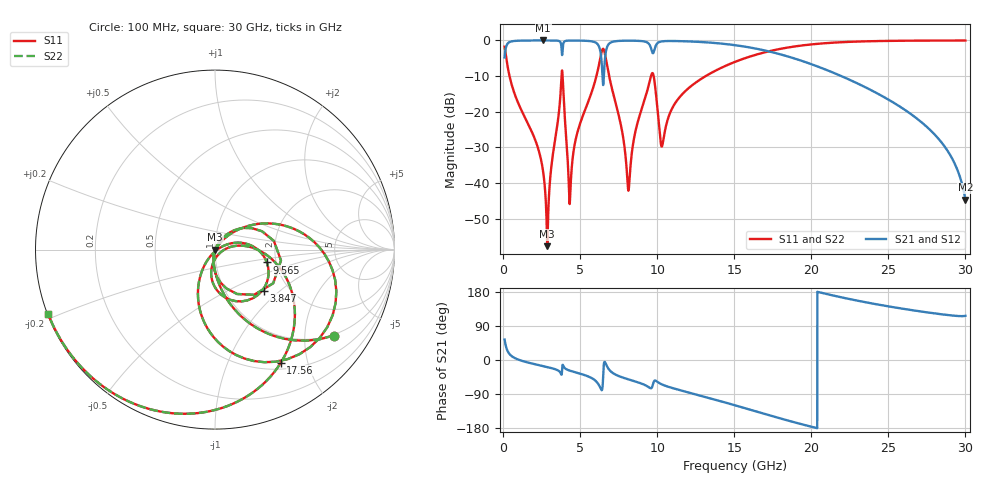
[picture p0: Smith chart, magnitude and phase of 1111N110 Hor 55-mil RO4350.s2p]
# GHz S MA R 50
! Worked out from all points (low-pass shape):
!   3201 points, 100 MHz to 30 GHz, reference 50 ohm
!   highest |S21| = -0.01 dB at 2.604 GHz (marker M1); lowest = -44.6 dB at 30 GHz (marker M2)
!   |S21| within 3 dB of the highest: 141.6 MHz to 3.807 GHz (3.665 GHz wide, 186 % of centre); 9.792 GHz to 17.18 GHz (7.388 GHz wide, 54.8 % of centre)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
!   lowest |S11| = -57.7 dB at 2.866 GHz (marker M3), VSWR 1.00, Z = 50.1 - j0.0687 ohm
!   |S11| at or under -10 dB: 419.5 MHz to 3.795 GHz (3.375 GHz wide, 160 % of centre); 6.882 GHz to 9.598 GHz (2.715 GHz wide, 33 % of centre); 9.772 GHz to 13.15 GHz (3.376 GHz wide, 29.5 % of centre)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
!   |S22| runs from -57.7 to 0.0 dB; largest |S21 - S12| = 0
!   S11 on the Smith chart (normalised r, x): 100 MHz: 0.97, -2.79; 3.847 GHz: 1.50, -0.79; 9.565 GHz: 1.78, -0.28; 17.56 GHz: 0.59, -1.58; 30 GHz: 0.00, -0.19
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0.1  0.8167 -35.9  0.5767 54.1  0.5767 54.1  0.8167 -35.9
0.585875  0.2293 -80.5  0.9728 9.4  0.9728 9.4  0.2293 -80.5
2.604125  0.01427 -101.9  0.9985 -16.2  0.9985 -16.2  0.01427 -101.9
2.86575  0.001308 -31.6  0.9984 -18.7  0.9984 -18.7  0.001308 -31.6
3.846844  0.3579 -40.1  0.6608 -16.8  0.6608 -16.8  0.3579 -40.1
4.332719  0.00527 -8.7  0.9945 -28.1  0.9945 -28.1  0.00527 -8.7
5.089563  0.07796 49.8  0.9923 -37.2  0.9923 -37.2  0.07796 49.8
6.15475  0.3876 21.1  0.875 -61.9  0.875 -61.9  0.3876 21.1
6.5285  0.7488 -51.2  0.2893 -16.0  0.2893 -16.0  0.7488 -51.2
6.874219  0.3226 -106.1  0.897 -25.0  0.897 -25.0  0.3226 -106.1
8.144969  0.007926 -42.1  0.9913 -51.3  0.9913 -51.3  0.007926 -42.1
9.565219  0.2977 -13.9  0.8185 -74.5  0.8185 -74.5  0.2977 -13.9
9.789469  0.3015 -70.6  0.7038 -56.5  0.7038 -56.5  0.3015 -70.6
10.06978  0.08501 -99.5  0.9326 -59.2  0.9326 -59.2  0.08501 -99.5
10.33141  0.03362 -31.6  0.9706 -64.9  0.9706 -64.9  0.03362 -31.6
11.59281  0.1732 6.5  0.9756 -80.9  0.9756 -80.9  0.1732 6.5
15.05  0.5004 -30.3  0.8576 -119.5  0.8576 -119.5  0.5004 -30.3
17.56347  0.7289 -59.8  0.6749 -149.2  0.6749 -149.2  0.7289 -59.8
20.03956  0.8807 -86.9  0.4615 -176.4  0.4615 -176.4  0.8807 -86.9
25.01978  0.9849 -129.2  0.1475 141.4  0.1475 141.4  0.9849 -129.2
28.44894  0.9956 -150.6  0.03725 120.6  0.03725 120.6  0.9956 -150.6
30  0.9963 -159.0  0.005869 116.6  0.005869 116.6  0.9963 -159.0
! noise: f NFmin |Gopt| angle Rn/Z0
0.1  0.000907  0.8025  2.681  0.0009523
3.417  0.01538  0.6341  21.92  0.007637
6.743  0.1175  0.8932  43.06  0.2076
10.06  0.1107  0.8397  62.35  0.1073
13.39  0.04048  0.5317  76.3  0.009971
16.7  0.0536  0.5763  89.53  0.0124
20.03  0.08273  0.6855  105.1  0.02
23.35  0.1509  0.8124  123  0.03965
26.67  0.3746  0.9204  141.5  0.1148
30  5.063  0.9932  159  7.032
